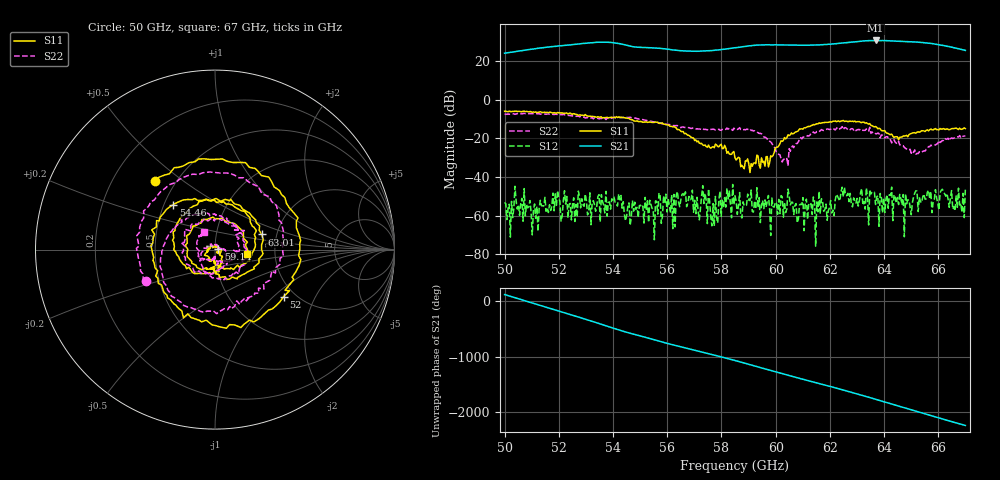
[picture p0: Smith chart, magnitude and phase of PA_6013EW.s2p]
!Agilent Technologies,E8361A,US42410132,A.06.03.05
!Agilent E8361A: A.06.03.05
!Date: Friday, July 11, 2008 13:05:18
!Correction: S11(Full 2 Port(1,2)) S21(Full 2 Port(1,2)) S12(Full 2 Port(1,2)) S22(Full 2 Port(1,2))
!S2P File: Measurements: S11, S21, S12, S22:
# Hz S  MA  R 50
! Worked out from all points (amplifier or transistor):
!   401 points, 50 GHz to 67 GHz, reference 50 ohm
!   highest |S21| = 30.9 dB at 63.69 GHz (marker M1)
!   |S21| within 3 dB of that: 58.94 GHz to 66.32 GHz (7.381 GHz wide, 11.8 % of centre)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
!   unconditionally stable (mu >= 1): start of sweep to end of sweep
!   at 52.8 GHz: K = 7.79, MAG = 30.7 dB, |S12| = -56.0 dB
!   at 58.5 GHz: K = 6.63, MAG = 27.2 dB, |S12| = -49.7 dB
!   at 67 GHz: K = 4.95, MAG = 25.9 dB, |S12| = -45.9 dB
!   S11 on the Smith chart (normalised r, x): 50 GHz: 0.39, +0.40; 52 GHz: 1.74, -1.16; 54.46 GHz: 0.56, +0.32; 59.14 GHz: 1.04, +0.01; 63.01 GHz: 1.67, +0.30; 67 GHz: 1.43, -0.07
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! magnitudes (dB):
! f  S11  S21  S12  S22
! 50 GHz  -5.9  24.3  -53.1  -7.5
! 51.06 GHz  -6.2  26.4  -57.6  -7.1
! 52 GHz  -6.7  28.0  -51.2  -7.8
! 52.85 GHz  -7.9  29.3  -51.3  -9.0
! 54.29 GHz  -9.0  29.1  -49.6  -9.2
! 54.46 GHz  -9.3  28.5  -62.7  -9.0
! 55.7 GHz  -12.1  26.8  -48.3  -12.0
! 56.2 GHz  -14.1  26.0  -66.8  -13.3
! 56.59 GHz  -16.4  25.5  -48.6  -14.0
! 57.14 GHz  -21.3  25.3  -57.9  -15.0
! 57.35 GHz  -23.7  25.4  -53.7  -15.4
! 57.65 GHz  -24.5  25.6  -65.3  -15.3
! 58.5 GHz  -30.1  27.1  -49.7  -15.3
! 59.14 GHz  -34.4  28.3  -57.9  -15.7
! 60.37 GHz  -20.2  28.5  -58.4  -31.2
! 61.35 GHz  -13.2  28.4  -59.4  -17.3
! 63.01 GHz  -11.3  30.3  -51.1  -15.5
! 63.69 GHz  -13.7  30.9  -54.3  -17.4
! 64.19 GHz  -17.9  30.7  -49.2  -19.5
! 65.26 GHz  -16.5  30.0  -57.9  -27.8
! 66.87 GHz  -15.2  26.2  -58.3  -18.7
! 67 GHz  -14.9  25.7  -45.9  -18.7
